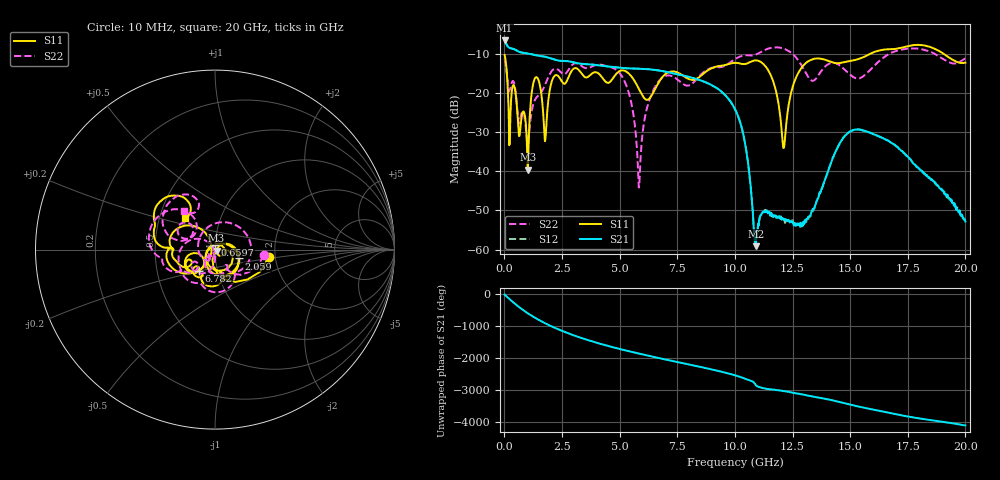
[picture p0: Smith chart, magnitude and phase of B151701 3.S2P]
!  2-Port S-parameters saved by WinCal
! VAR MeasName=S-Parameters (CALIBRATED_DATA) read from VNA (N5244A)
! VAR MeasDate=2015-12-24 19:08:33
! VAR NAME=B151701 3
! VAR FILENAME=B151701 3.S2P
! VAR DATE=2015-12-24 19:08:33
! VAR PHYS_PORTS=1,3
# Hz S DB R 50
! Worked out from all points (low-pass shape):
!   801 points, 10 MHz to 20 GHz, reference 50 ohm
!   highest |S21| = -6.68 dB at 10 MHz (marker M1); lowest = -59.1 dB at 10.9 GHz (marker M2)
!   |S21| within 3 dB of the highest: start of sweep to 693.2 MHz
!   lowest |S11| = -39.6 dB at 1.01 GHz (marker M3), VSWR 1.02, Z = 50.9 - j0.577 ohm
!   |S11| at or under -10 dB: start of sweep to 15.9 GHz; 19.04 GHz to end of sweep
!   |S22| runs from -44.2 to -8.4 dB; largest |S21 - S12| = 0.00089
!   S11 on the Smith chart (normalised r, x): 10 MHz: 1.85, -0.17; 659.7 MHz: 1.00, +0.06; 2.059 GHz: 1.30, -0.13; 6.782 GHz: 0.81, -0.20; 20 GHz: 0.68, +0.25
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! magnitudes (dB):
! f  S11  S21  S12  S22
! 10 MHz  -10.4  -6.7  -6.7  -11.2
! 209.9 MHz  -33.4  -8.5  -8.5  -19.7
! 659.7 MHz  -31.0  -9.6  -9.6  -27.6
! 1.01 GHz  -39.6  -10.0  -10.0  -32.9
! 1.309 GHz  -16.5  -10.4  -10.4  -22.0
! 1.759 GHz  -32.4  -10.8  -10.8  -18.1
! 2.059 GHz  -17.1  -11.3  -11.3  -14.4
! 3.358 GHz  -15.2  -12.6  -12.6  -13.2
! 5.132 GHz  -14.3  -13.7  -13.7  -16.1
! 5.832 GHz  -19.0  -13.9  -13.9  -44.2
! 6.682 GHz  -17.5  -14.3  -14.3  -17.2
! 6.782 GHz  -16.6  -14.4  -14.4  -16.5
! 10.01 GHz  -12.4  -24.2  -24.2  -11.4
! 10.45 GHz  -12.7  -33.4  -33.3  -10.4
! 10.9 GHz  -11.8  -59.1  -58.7  -10.3
! 11.65 GHz  -17.0  -51.7  -51.1  -8.5
! 12.1 GHz  -34.1  -52.1  -52.4  -8.7
! 12.6 GHz  -16.8  -53.8  -53.2  -10.7
! 13.35 GHz  -11.5  -50.0  -50.7  -16.9
! 14.85 GHz  -12.1  -30.5  -30.5  -14.6
! 16.68 GHz  -8.9  -32.3  -32.3  -10.2
! 20 GHz  -12.3  -52.8  -52.4  -11.2
